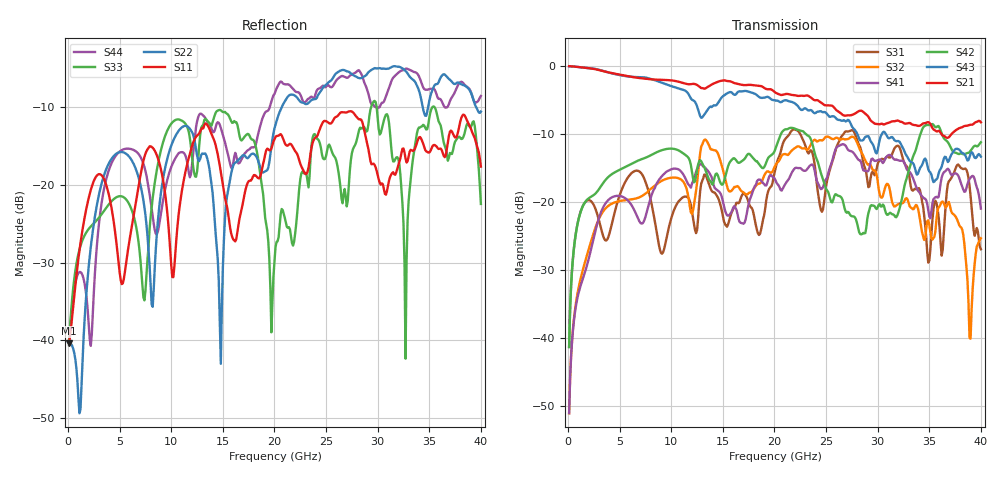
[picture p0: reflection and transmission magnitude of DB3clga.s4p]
! ADC12DJ3200QML-SP
! 196-pin ZMX package
! CLGA Ceramic Package without columns (ceramic land grid array)
! Texas Instruments 4/21/2021
! Single-ended  S-parameters
! PORT#  PORT_NAME  NET_NAME
! PORT1:  DAxN.DIEBUMP DAxN
! PORT2:  DAxN.BGA  DAxN
! PORT3:  DAxP.DIEBUMP DAxP
! PORT4:  DAxP.BGA  DAxP
! Touchstone Ver. 1.0
! Number of ports is 4
# Hz	S	MA	R	50.000000
! SCATTERING PARAMETERS  :
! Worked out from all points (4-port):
!   400 points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, 100 MHz to 40 GHz, reference 50 ohm
!   strongest paths, dB at 100 MHz, 10.1 GHz, 20.1 GHz, 30.1 GHz, 40 GHz:
!     S21: -0.1, -2.2, -4.0, -8.6, -8.3
!     S43: -0.1, -3.1, -5.1, -11.6, -13.4
!     S42: -41.4, -12.2, -12.2, -20.5, -11.3
!     S41: -51.1, -15.2, -16.9, -13.9, -21.0
!     S32: -51.1, -16.5, -14.6, -18.2, -25.4
!     S31: -41.4, -21.9, -15.2, -14.1, -27.0
!   lowest |S11| = -40.4 dB at 100 MHz (marker M1), VSWR 1.02, Z = 51 + j0.0403 ohm
!   |S11| at or under -10 dB: start of sweep to end of sweep
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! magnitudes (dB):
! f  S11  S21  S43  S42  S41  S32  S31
! 100 MHz  -40.4  -0.1  -0.1  -41.4  -51.1  -51.1  -41.4
! 13.2 GHz  -12.3  -3.4  -7.2  -14.9  -14.9  -10.9  -16.0
! 14.8 GHz  -18.3  -2.2  -4.9  -17.4  -18.9  -14.2  -20.7
! 19.7 GHz  -15.3  -3.5  -5.0  -13.2  -16.2  -15.8  -17.7
! 23.8 GHz  -14.2  -5.0  -6.9  -12.3  -14.9  -11.0  -13.7
! 32.7 GHz  -16.6  -8.5  -13.0  -17.1  -14.8  -19.6  -14.6
! 40 GHz  -17.6  -8.3  -13.4  -11.3  -21.0  -25.4  -27.0
